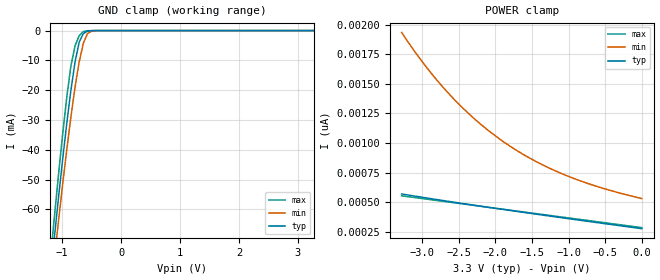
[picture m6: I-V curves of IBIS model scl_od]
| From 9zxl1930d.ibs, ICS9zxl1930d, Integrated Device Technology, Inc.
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|   Model scl_od
[Model]  scl_od
Model_type Input
Polarity   Non-Inverting
Vinl =   0.8000V
Vinh =   2.0000V
C_comp   1.3700pF   1.3700pF   1.3700pF
[Temperature Range]   25.0000   85.0000   -40.0000
[Voltage Range]   3.3000V   3.1350V   3.4650V
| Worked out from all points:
|   GND clamp passes 1 mA (typ) near -0.64 V on its own axis
[GND_clamp]
|Voltage   I(typ)   I(min)   I(max)
-3.3V     -543.2mA   -525.9mA   -564.4mA
-1.2V     -83.07mA   -89.44mA   -77.25mA
-1.13V    -69.33mA   -76.46mA   -62.52mA
-1.06V    -56.02mA   -63.82mA   -48.3mA
-920mV    -31.14mA   -39.94mA   -22.33mA
-850mV    -20.04mA   -28.97mA   -11.85mA
-780mV    -10.54mA   -19.02mA   -5.158mA
-710mV    -3.899mA   -10.54mA   -1.704mA
-640mV    -1.024mA   -4.284mA   -353.9uA
-570mV    -215.4uA   -1.064mA   -49.93uA
-430mV    -5.637uA   -33.74uA   -408.6nA
3.28V     273.7pA    551.6pA    269pA
[POWER_clamp]
|Voltage   I(typ)   I(min)   I(max)
-3.28V    568.6pA    1.935nA    553.1pA
-3.12V    552.7pA    1.789nA    540pA
-2.92V    533.2pA    1.624nA    523.5pA
-2.72V    514pA      1.475nA    507.2pA
-2.6V     502.6pA    1.393nA    497.4pA
-2.4V     483.9pA    1.269nA    480.9pA
-2.24V    469.1pA    1.179nA    467.8pA
-1.88V    436.6pA    1.006nA    438.3pA
-1.52V    404.7pA    868.3pA    408.8pA
-1.08V    366.6pA    737.3pA    372.7pA
-560mV    322.3pA    622.4pA    330.1pA
0V        275.4pA    529.9pA    284.1pA
